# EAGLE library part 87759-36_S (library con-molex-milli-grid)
HEADER
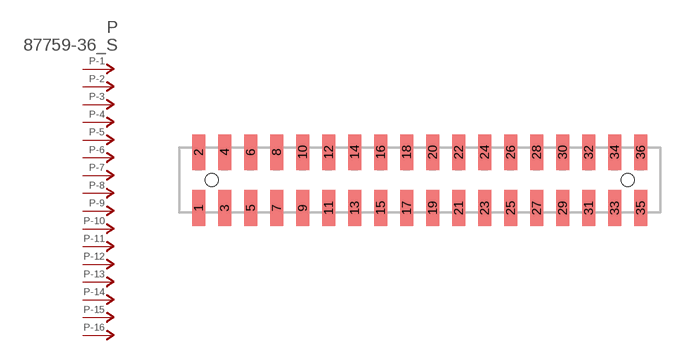
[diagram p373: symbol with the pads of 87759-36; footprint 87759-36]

Designator prefix P; gates -1=P-NV -2=P-N -3=P-N -4=P-N -5=P-N -6=P-N -7=P-N -8=P-N -9=P-N -10=P-N -11=P-N -12=P-N -13=P-N -14=P-N -15=P-N -16=P-N -17=P-N -18=P-N -19=P-N -20=P-N -21=P-N -22=P-N -23=P-N -24=P-N -25=P-N -26=P-N -27=P-N -28=P-N -29=P-N -30=P-N -31=P-N -32=P-N -33=P-N -34=P-N -35=P-N -36=P-N

## 87759-36_S  [87759-36]
1  -1:P  pas
2  -2:P  pas
3  -3:P  pas
4  -4:P  pas
5  -5:P  pas
6  -6:P  pas
7  -7:P  pas
8  -8:P  pas
9  -9:P  pas
10  -10:P  pas
11  -11:P  pas
12  -12:P  pas
13  -13:P  pas
14  -14:P  pas
15  -15:P  pas
16  -16:P  pas
17  -17:P  pas
18  -18:P  pas
19  -19:P  pas
20  -20:P  pas
21  -21:P  pas
22  -22:P  pas
23  -23:P  pas
24  -24:P  pas
25  -25:P  pas
26  -26:P  pas
27  -27:P  pas
28  -28:P  pas
29  -29:P  pas
30  -30:P  pas
31  -31:P  pas
32  -32:P  pas
33  -33:P  pas
34  -34:P  pas
35  -35:P  pas
36  -36:P  pas

## Footprint 87759-36 (pad centres in mm)
HEADER SMD Dual Row, Vertical
smd 1 x 2.75: 1 -17,-2.15; 2 -17,2.15; 3 -15,-2.15; 4 -15,2.15; 5 -13,-2.15; 6 -13,2.15; 7 -11,-2.15; 8 -11,2.15; 9 -9,-2.15; 10 -9,2.15; 11 -7,-2.15; 12 -7,2.15; 13 -5,-2.15; 14 -5,2.15; 15 -3,-2.15; 16 -3,2.15; 17 -1,-2.15; 18 -1,2.15; 19 1,-2.15; 20 1,2.15; 21 3,-2.15; 22 3,2.15; 23 5,-2.15; 24 5,2.15; 25 7,-2.15; 26 7,2.15; 27 9,-2.15; 28 9,2.15; 29 11,-2.15; 30 11,2.15; 31 13,-2.15; 32 13,2.15; 33 15,-2.15; 34 15,2.15; 35 17,-2.15; 36 17,2.15
hole 1 at -16,0
hole 1 at 16,0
